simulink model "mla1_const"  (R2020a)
settings: Solver=ode5  StartTime=0.0  StopTime=2  FixedStep=0.0001  RelTol=1e-4  EnableMultiTasking=on
PreLoadFcn:
  | MLA_Sensor1 = load('mla_sensor1.dat');
libraries: libmla x1

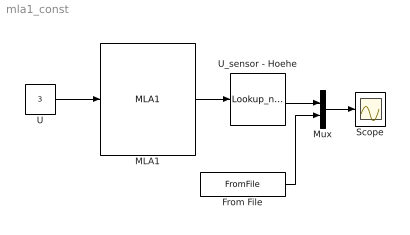
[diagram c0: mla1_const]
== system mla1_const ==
  From File : FromFile  FileName=mla_const.mat  SampleTime=0
  MLA1 : libmla/MLA1  g=9.81  m=0.125  d_l=0.42  a=40691  b=0.0687  N=4.282
  Mux : Mux  Inputs=2
  Scope : Scope
  U : Constant  Value=3
  U_sensor - Hoehe : Lookup_n-D  NumberOfTableDimensions=1  BreakpointsForDimension1=MLA_Sensor1(:,1)  Table=MLA_Sensor1(:,2)  RndMeth=Simplest
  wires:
  MLA1/1 -> U_sensor - Hoehe/1
  U/1 -> MLA1/1
  U_sensor - Hoehe/1 -> Mux/1
  Mux/1 -> Scope/1
  From File/1 -> Mux/2
